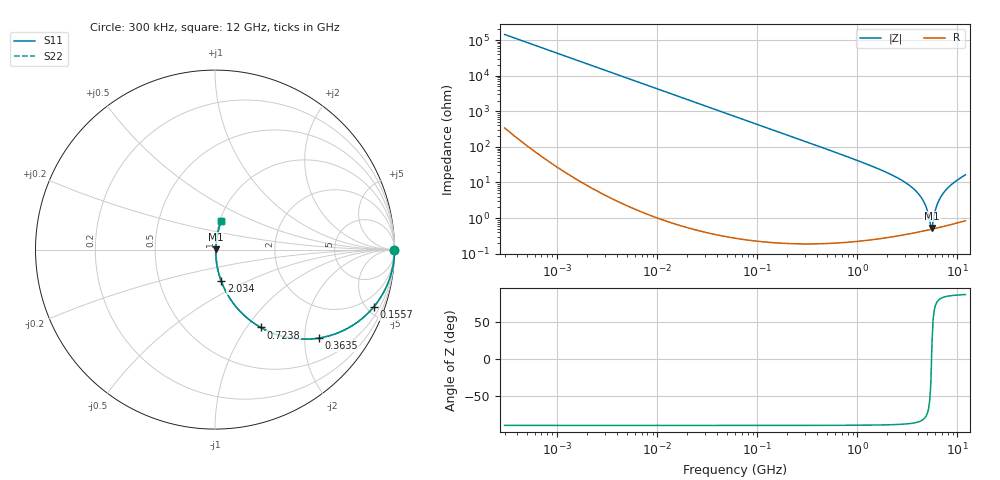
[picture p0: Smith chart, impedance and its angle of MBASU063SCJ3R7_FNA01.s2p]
! MBASU063SCJ3R7_FNA01  S-PARAMETER MODEL  ( General Type )
! Model Generated by TAIYO YUDEN Corporation (http://www.ty-top.com)
! Version 1.0
! TAIYO YUDEN Control No. 130801
! Copyright(c) 2013 TAIYO YUDEN CO.,LTD. All Rights Reserved.
! Product Description (link to TY-COMPAS)
! https://ds.yuden.co.jp/TYCOMPAS/or/detail?pn=MBASU063SCJ3R7CFNA01&u=M
! Products Name : Multilayer Ceramic Capacitors
! Characteristics :
!  Capacitance : 3.7 pF , Rated Voltage : 50V , TCC : CJ / C0J
!  Case Size : 0.6 x 0.3 / 0.024 x 0.012 [mm/inch] , Thickness : 0.3 / 0.012 [mm/inch]
!  (Conditions: Temperature = 25 degC , DC Bias Current/Voltage = 0A / 0V)
! External Node Assignments :
!  1  o---| |---o  2
! GND o---------o GND
! Frequency Range : 0.3MHz  -  12000MHz  [ 401 STEP ]
# MHz S RI R 50
! Freq[MHz].  S11 Real  S11 Imag  S21 Real  S21 Imag  S12 Real  S12 Imag  S22 Real  S22 Imag
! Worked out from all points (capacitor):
!   401 points, 300 kHz to 12 GHz, reference 50 ohm
!   read as one part in series: C = 3.71 pF near 316.3 kHz
!   lowest |Z| = 529 mohm at 5.566 GHz (marker M1)
!   series resonance near 5.51 GHz, so ESL is about 230 pH
!   S11 on the Smith chart (normalised r, x): 300 kHz: open; 155.7 MHz: 1.00, -5.51; 363.5 MHz: 1.00, -2.35; 723.8 MHz: 1.00, -1.17; 2.034 GHz: 1.01, -0.37; 12 GHz: 1.02, +0.33
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0.3  1 -0.000699  2.15e-06 0.000699  2.15e-06 0.000699  1 -0.000699
1.769972  1 -0.00412  1.87e-05 0.00412  1.87e-05 0.00412  1 -0.00412
10.44266  0.9994 -0.0243  0.000597 0.0243  0.000597 0.0243  0.9994 -0.0243
60  0.9808 -0.1371  0.0192 0.1371  0.0192 0.1371  0.9808 -0.1371
155.7172  0.8834 -0.3206  0.1166 0.3206  0.1166 0.3206  0.8834 -0.3206
353.9943  0.5932 -0.4905  0.4068 0.4905  0.4068 0.4905  0.5932 -0.4905
363.4975  0.5803 -0.4927  0.4197 0.4927  0.4197 0.4927  0.5803 -0.4927
723.8279  0.2544 -0.4338  0.7456 0.4338  0.7456 0.4338  0.2544 -0.4338
1166.079  0.1118 -0.3118  0.8882 0.3118  0.8882 0.3118  0.1118 -0.3118
2033.931  0.0348 -0.1757  0.9652 0.1757  0.9652 0.1757  0.0348 -0.1757
2088.533  0.0328 -0.17  0.9672 0.17  0.9672 0.17  0.0328 -0.17
3026.31  0.0131 -0.0977  0.9869 0.0977  0.9869 0.0977  0.0131 -0.0977
3944.255  0.00678 -0.0529  0.9932 0.0529  0.9932 0.0529  0.00678 -0.0529
4623.766  0.00512 -0.0276  0.9949 0.0276  0.9949 0.0276  0.00512 -0.0276
4875.354  0.00487 -0.0194  0.9951 0.0194  0.9951 0.0194  0.00487 -0.0194
5278.635  0.00477 -0.00711  0.9952 0.00711  0.9952 0.00711  0.00477 -0.00711
5565.855  0.00488 0.00197  0.9951 -0.00197  0.9951 -0.00197  0.00488 0.00197
5715.274  0.005 0.00672  0.995 -0.00672  0.995 -0.00672  0.005 0.00672
6354.153  0.00597 0.0256  0.994 -0.0256  0.994 -0.0256  0.00597 0.0256
7254.098  0.00833 0.0501  0.9917 -0.0501  0.9917 -0.0501  0.00833 0.0501
8966.534  0.0152 0.0911  0.9848 -0.0911  0.9848 -0.0911  0.0152 0.0911
12000  0.0339 0.1573  0.9661 -0.1573  0.9661 -0.1573  0.0339 0.1573
